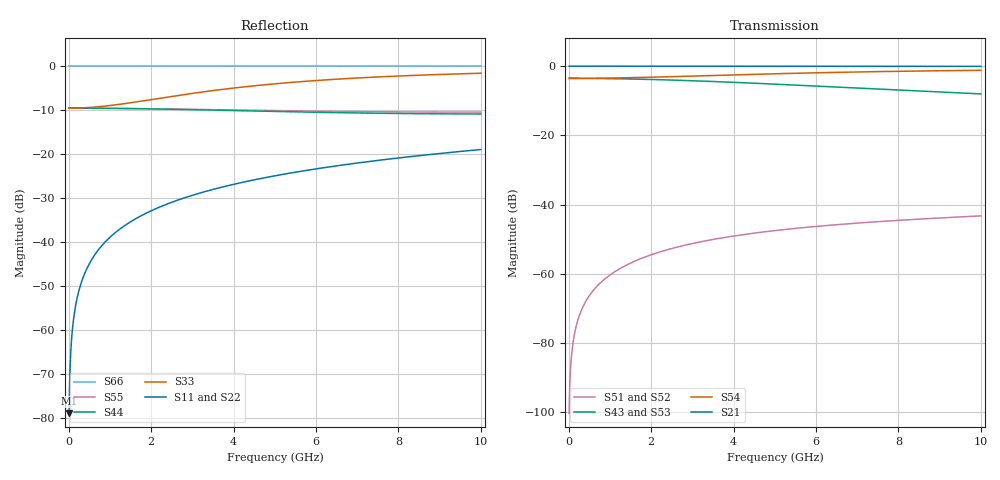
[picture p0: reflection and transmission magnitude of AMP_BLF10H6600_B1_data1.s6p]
! Created Tue Feb  9 11:55:40 2010
# ghz S ma R 50
! 6 Port Network Data from SP1.SP block
! freq  magS11  angS11  magS12  angS12  magS13  angS13  magS14  angS14
!  magS15  angS15  magS16  angS16
!  magS21  angS21  magS22  angS22
!  magS23  angS23  magS24  angS24  magS25  angS25  magS26  angS26
!  magS31  angS31  magS32  angS32  magS33  angS33  magS34  angS34
!  magS35  angS35  magS36  angS36
!  magS41  angS41  magS42  angS42
!  magS43  angS43  magS44  angS44  magS45  angS45  magS46  angS46
!  magS51  angS51  magS52  angS52  magS53  angS53  magS54  angS54
!  magS55  angS55  magS56  angS56
!  magS61  angS61  magS62  angS62
!  magS63  angS63  magS64  angS64  magS65  angS65  magS66  angS66
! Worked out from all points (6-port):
!   1000 points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, 10 MHz to 10 GHz, reference 50 ohm
!   strongest paths, dB at 10 MHz, 2.51 GHz, 5.01 GHz, 7.51 GHz, 10 GHz:
!     S21: 0.0, 0.0, 0.0, 0.0, -0.1
!     S54: -3.5, -3.0, -2.2, -1.6, -1.2
!     S43: -3.5, -4.0, -5.2, -6.6, -8.0
!     S53: -3.5, -4.0, -5.3, -6.8, -8.3
!     S51: -100.2, -52.6, -47.5, -44.9, -43.2
!     S52: -100.2, -52.6, -47.5, -44.9, -43.2
!   lowest |S11| = -78.9 dB at 10 MHz (marker M1), VSWR 1.00, Z = 50 + j0.0114 ohm
!   |S11| at or under -10 dB: start of sweep to end of sweep
